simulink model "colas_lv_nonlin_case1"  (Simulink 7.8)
settings: Solver=ode45  SolverMode=SingleTasking  StartTime=0  StopTime=130  MaxStep=1  RelTol=1e-5  AbsTol=1e-5

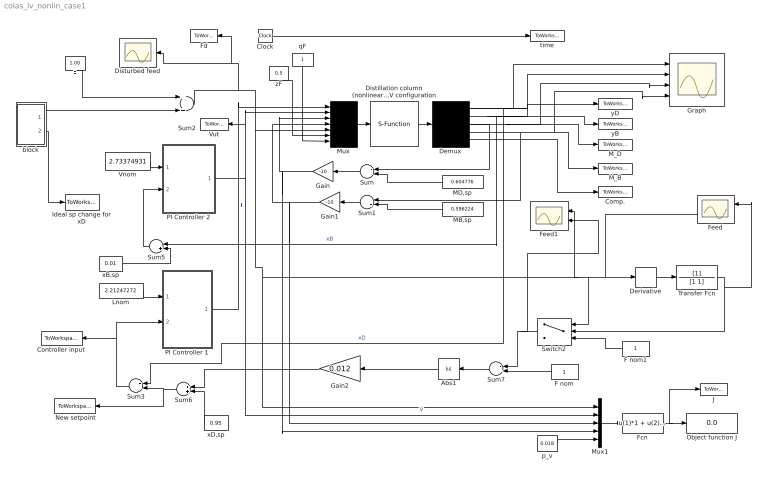
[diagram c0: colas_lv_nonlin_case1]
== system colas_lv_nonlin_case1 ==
  " New setpoint" : ToWorkspace  VariableName=setp  SaveFormat=Structure With Time
  Abs1 : Abs
  Clock : Clock
  Comp. : ToWorkspace  VariableName=Comp  SaveFormat=Structure With Time
  Controller input : ToWorkspace  VariableName=inp  SaveFormat=Structure With Time
  Demux : Demux  Outputs=[1,1,1,1,82]
  Derivative : Derivative
  Distillation column (nonlinear)  LV configuration : S-Function  FunctionName=scolas_orig  EnableBusSupport=off
  Disturbed feed : Scope
  F : Constant  Value=1.00
  F nom : Constant
  F nom1 : Constant
  Fcn : Fcn  Expr=u(1)*1 + u(2)*u(5) - u(3)*1-u(4)*2
  Fd : ToWorkspace  VariableName=Fd  SaveFormat=Structure With Time
  Feed : Scope  NumInputPorts=2
  Feed1 : Scope  NumInputPorts=2
  Gain : Gain  Gain=-10
  Gain1 : Gain  Gain=-10
  Gain2 : Gain  Gain=0.012
  Graph : Scope  NumInputPorts=4
  Ideal sp change for xD : ToWorkspace  VariableName=idealsp  SaveFormat=Structure With Time
  J : ToWorkspace  VariableName=J  SaveFormat=Structure With Time
  Lnom : Constant  Value=2.21247272
  MB,sp : Constant  Value=0.596224
  MD,sp : Constant  Value=0.604776
  M_B : ToWorkspace  VariableName=y4  SaveFormat=Structure With Time
  M_D : ToWorkspace  VariableName=y3  SaveFormat=Structure With Time
  Mux : Mux  Inputs=7
  Mux1 : Mux  Inputs=5
  Object function J : Display
  PI Controller 1 : Subsystem
  PI Controller 2 : Subsystem
  Sum{,1,3,5,7} (5 alike) : Sum  Inputs=-+
  Sum2 : Sum
  Sum6 : Sum
  Switch2 : Switch  Criteria=u2 ~= 0
  Transfer Fcn : TransferFcn  Denominator=[1 1]
  Vnom : Constant  Value=2.73374931
  Vut : ToWorkspace  VariableName=Vut  SaveFormat=Structure With Time
  block : Subsystem
  p_v : Constant  Value=0.018
  qF : Constant
  time : ToWorkspace  VariableName=t  SaveFormat=Array
  xB,sp : Constant  Value=0.01
  xD,sp : Constant  Value=0.95
  yB : ToWorkspace  VariableName=y2  SaveFormat=Structure With Time
  yD : ToWorkspace  VariableName=y1  SaveFormat=Structure With Time
  zF : Constant  Value=0.5
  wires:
  qF/1 -> Mux/7
  Demux/1 -> yD/1, Sum3/1, Graph/1  "xD"
  Gain1/1 -> Mux/4, Mux1/3
  Sum1/1 -> Gain1/1
  MB,sp/1 -> Sum1/2
  Demux/4 -> Sum1/1, M_B/1, Graph/4
  Demux/3 -> Sum/1, Graph/3, M_D/1
  Gain/1 -> Mux/3, Mux1/4
  MD,sp/1 -> Sum/2
  Sum/1 -> Gain/1
  Mux/1 -> Distillation column (nonlinear)  LV configuration/1
  Distillation column (nonlinear)  LV configuration/1 -> Demux/1
  Clock/1 -> time/1
  zF/1 -> Mux/6
  Demux/5 -> Comp./1
  Sum3/1 -> PI Controller 1/2(SP error), Controller input/1
  Sum5/1 -> PI Controller 2/2(SP error)
  Sum2/1 -> Disturbed feed/1, Fd/1, Mux/5, Mux1/1, Feed1/1, Derivative/1, Feed/2, Switch2/1
  p_v/1 -> Mux1/5
  Fcn/1 -> Object function J/1, J/1
  Mux1/1 -> Fcn/1
  Lnom/1 -> PI Controller 1/1(Nom. value)
  PI Controller 1/1(L) -> Mux/1  "L"
  Vnom/1 -> PI Controller 2/1(Nom. value)
  PI Controller 2/1(V) -> Mux1/2, Mux/2, Vut/1  "V"
  xB,sp/1 -> Sum5/2
  Transfer Fcn/1 -> Switch2/2, Feed/1
  Switch2/1 -> Sum7/1, Feed1/2
  F nom/1 -> Sum7/2
  Sum7/1 -> Abs1/1
  Abs1/1 -> Gain2/1
  F/1 -> Sum2/1
  xD,sp/1 -> Sum6/2
  Demux/2 -> Sum5/1, yB/1, Graph/2  "xB"
  Derivative/1 -> Transfer Fcn/1
  F nom1/1 -> Switch2/3
  block/2(Out2) -> Ideal sp change for xD/1
  block/1(Out1) -> Sum2/2
  Gain2/1 -> Sum6/1
  Sum6/1 -> Sum3/2, " New setpoint"/1

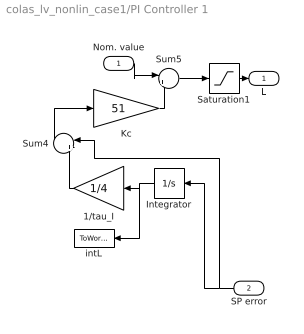
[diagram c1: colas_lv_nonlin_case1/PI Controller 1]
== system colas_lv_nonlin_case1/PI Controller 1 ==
  Nom. value : Inport
  SP error : Inport  Port=2
  1/tau_I : Gain  Gain=1/4
  Integrator : Integrator  InitialCondition=0.0004
  Kc : Gain  Gain=51
  Saturation1 : Saturate  UpperLimit=inf  LowerLimit=0
  Sum4 : Sum  Inputs=|++
  Sum5 : Sum  Inputs=|++
  intL : ToWorkspace  VariableName=intL  SaveFormat=Array
  L : Outport
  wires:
  SP error/1 -> Sum4/1, Integrator/1
  Integrator/1 -> 1/tau_I/1, intL/1
  1/tau_I/1 -> Sum4/2
  Sum4/1 -> Kc/1
  Kc/1 -> Sum5/2
  Nom. value/1 -> Sum5/1
  Saturation1/1 -> L/1
  Sum5/1 -> Saturation1/1

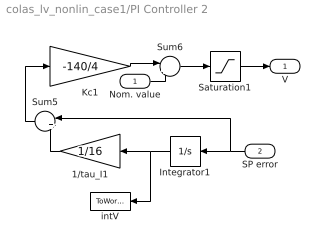
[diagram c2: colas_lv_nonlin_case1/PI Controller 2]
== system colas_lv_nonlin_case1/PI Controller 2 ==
  Nom. value : Inport
  SP error : Inport  Port=2
  1/tau_I1 : Gain  Gain=1/16
  Integrator1 : Integrator  InitialCondition=-0.0002
  Kc1 : Gain  Gain=-140/4
  Saturation1 : Saturate  UpperLimit=inf  LowerLimit=0
  Sum5 : Sum  Inputs=|++
  Sum6 : Sum  Inputs=|++
  intV : ToWorkspace  VariableName=intV  SaveFormat=Array
  V : Outport
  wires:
  SP error/1 -> Sum5/1, Integrator1/1
  Integrator1/1 -> 1/tau_I1/1, intV/1
  1/tau_I1/1 -> Sum5/2
  Sum5/1 -> Kc1/1
  Kc1/1 -> Sum6/1
  Nom. value/1 -> Sum6/2
  Sum6/1 -> Saturation1/1
  Saturation1/1 -> V/1

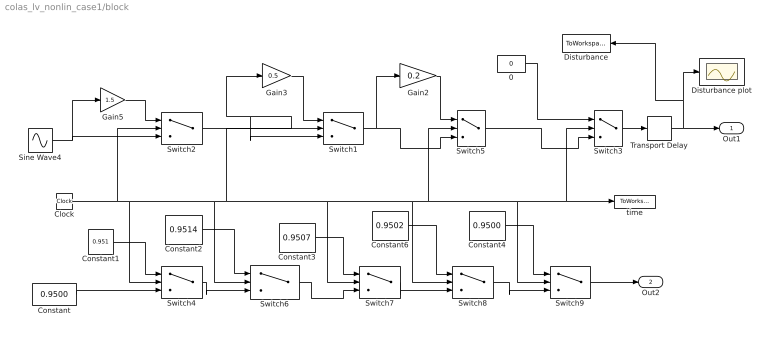
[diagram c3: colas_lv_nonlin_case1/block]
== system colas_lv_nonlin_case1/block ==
  0 : Constant  Value=0
  Clock : Clock
  Constant : Constant  Value=0.9500
  Constant1 : Constant  Value=0.951
  Constant2 : Constant  Value=0.9514
  Constant3 : Constant  Value=0.9507
  Constant4 : Constant  Value=0.9500
  Constant6 : Constant  Value=0.9502
  Disturbance : ToWorkspace  VariableName=wa  SaveFormat=Structure With Time
  Disturbance plot : Scope
  Gain2 : Gain  Gain=0.2
  Gain3 : Gain  Gain=0.5
  Gain5 : Gain  Gain=1.5
  Sine Wave4 : Sin  Amplitude=0.2  SampleTime=0
  Switch1 : Switch  Criteria=u2 > Threshold  Threshold=62.9
  Switch2 : Switch  Criteria=u2 > Threshold  Threshold=28.3
  Switch3 : Switch  Criteria=u2 > Threshold  Threshold=106.8
  Switch4 : Switch  Criteria=u2 > Threshold  Threshold=10
  Switch5 : Switch  Criteria=u2 > Threshold  Threshold=87
  Switch6 : Switch  Criteria=u2 > Threshold  Threshold=38.3
  Switch7 : Switch  Criteria=u2 > Threshold  Threshold=72.9
  Switch8 : Switch  Criteria=u2 > Threshold  Threshold=97
  Switch9 : Switch  Criteria=u2 > Threshold  Threshold=116.8
  Transport Delay : TransportDelay  DelayTime=10
  time : ToWorkspace  VariableName=t1  SaveFormat=Array
  Out1 : Outport
  Out2 : Outport  Port=2
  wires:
  Clock/1 -> Switch2/2, Switch4/2, Switch1/2, Switch7/2, Switch5/2, time/1, Switch3/2, Switch9/2, Switch8/2, Switch6/2
  Switch2/1 -> Gain3/1, Switch1/3
  Gain5/1 -> Switch2/1
  Gain3/1 -> Switch1/1
  Sine Wave4/1 -> Switch2/3, Gain5/1
  0/1 -> Switch3/1
  Transport Delay/1 -> Out1/1, Disturbance plot/1, Disturbance/1
  Switch3/1 -> Transport Delay/1
  Switch1/1 -> Switch5/3, Gain2/1
  Switch5/1 -> Switch3/3
  Gain2/1 -> Switch5/1
  Constant/1 -> Switch4/3
  Constant1/1 -> Switch4/1
  Switch4/1 -> Switch6/3
  Constant2/1 -> Switch6/1
  Switch6/1 -> Switch7/3
  Constant3/1 -> Switch7/1
  Switch7/1 -> Switch8/3
  Constant6/1 -> Switch8/1
  Constant4/1 -> Switch9/1
  Switch8/1 -> Switch9/3
  Switch9/1 -> Out2/1
